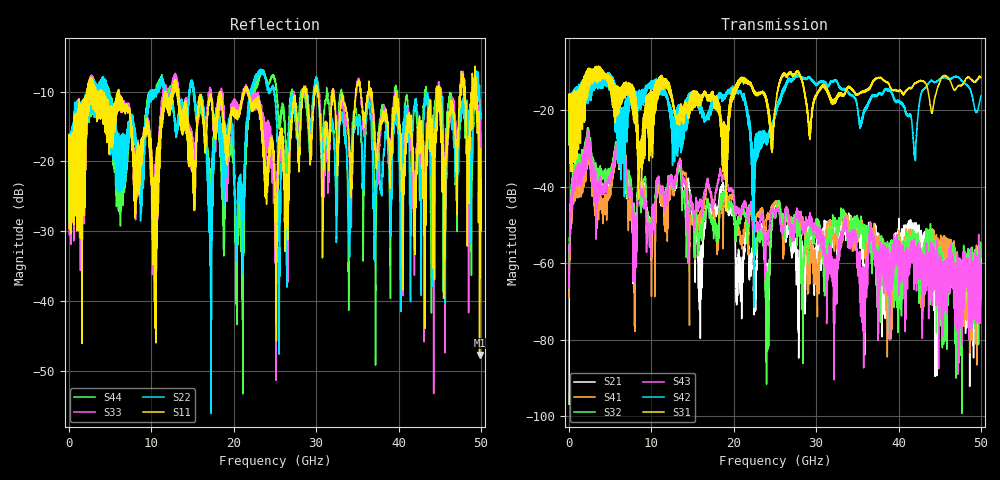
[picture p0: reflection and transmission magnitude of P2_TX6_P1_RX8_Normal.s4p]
!Keysight Technologies,N5225B,MY57041031,A.13.20.10
!Date: Friday, May 31, 2019 11:27:03
!Correction: S11(Full 4 Port(1,2,3,4))
!S12(Full 4 Port(1,2,3,4))
!S13(Full 4 Port(1,2,3,4))
!S14(Full 4 Port(1,2,3,4))
!S21(Full 4 Port(1,2,3,4))
!S22(Full 4 Port(1,2,3,4))
!S23(Full 4 Port(1,2,3,4))
!S24(Full 4 Port(1,2,3,4))
!S31(Full 4 Port(1,2,3,4))
!S32(Full 4 Port(1,2,3,4))
!S33(Full 4 Port(1,2,3,4))
!S34(Full 4 Port(1,2,3,4))
!S41(Full 4 Port(1,2,3,4))
!S42(Full 4 Port(1,2,3,4))
!S43(Full 4 Port(1,2,3,4))
!S44(Full 4 Port(1,2,3,4))
!S4P File: Measurements: <S11,S12,S13,S14>,
!<S21,S22,S23,S24>,
!<S31,S32,S33,S34>,
!<S41,S42,S43,S44>:
# Hz S  dB  R 50.0
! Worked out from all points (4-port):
!   5000 points, 10 MHz to 50 GHz, reference 50 ohm
!   strongest paths, dB at 10 MHz, 12.51 GHz, 25.01 GHz, 37.51 GHz, 50 GHz:
!     S31: -19.4, -16.7, -19.9, -11.6, -11.4
!     S42: -19.4, -24.1, -21.9, -15.8, -16.2
!     S43: -61.0, -37.2, -48.2, -78.5, -65.1
!     S32: -66.8, -37.7, -47.4, -65.4, -63.4
!     S41: -60.3, -40.0, -44.6, -55.6, -60.9
!     S21: -96.9, -39.3, -44.8, -57.5, -60.1
!   lowest |S11| = -47.8 dB at 49.84 GHz (marker M1), VSWR 1.01, Z = 50 + j0.407 ohm
!   |S11| at or under -10 dB: 6.028 GHz to 11.67 GHz (5.642 GHz wide, 63.8 % of centre); 21.74 GHz to 28.38 GHz (6.637 GHz wide, 26.5 % of centre); 36.76 GHz to 44.63 GHz (7.865 GHz wide, 19.3 % of centre)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
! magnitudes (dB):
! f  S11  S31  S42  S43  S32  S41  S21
! 10 MHz  -19.5  -19.4  -19.4  -61.0  -66.8  -60.3  -96.9
! 2.35 GHz  -13.3  -14.8  -16.7  -25.4  -24.7  -25.4  -24.9
! 20.37 GHz  -13.0  -13.1  -14.6  -46.0  -49.1  -51.9  -69.5
! 24.04 GHz  -22.0  -18.5  -28.3  -53.1  -80.3  -47.4  -66.4
! 25.43 GHz  -21.9  -13.6  -17.5  -45.9  -44.2  -45.7  -44.0
! 49.84 GHz  -47.8  -11.2  -17.8  -63.5  -58.4  -74.9  -70.7
! 50 GHz  -22.5  -11.4  -16.2  -65.1  -63.4  -60.9  -60.1
